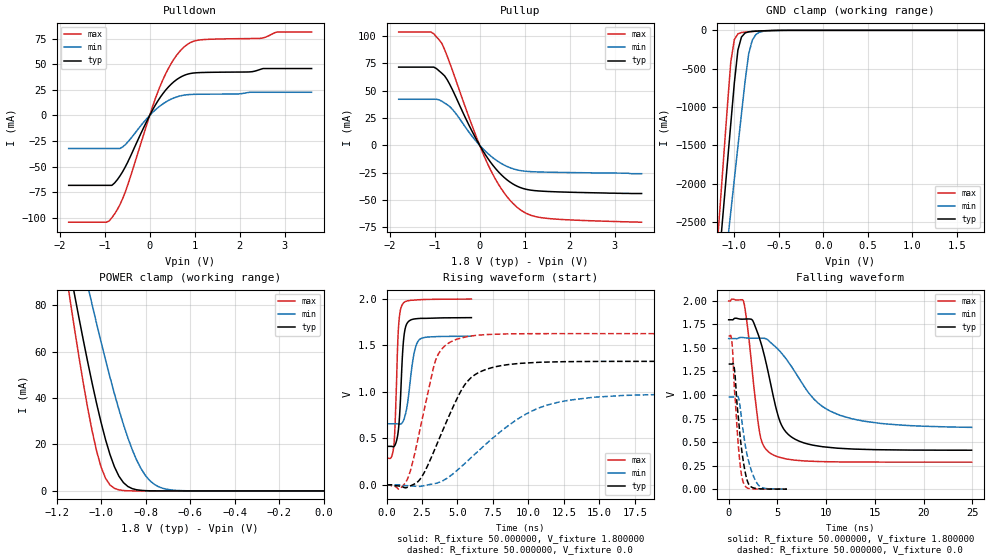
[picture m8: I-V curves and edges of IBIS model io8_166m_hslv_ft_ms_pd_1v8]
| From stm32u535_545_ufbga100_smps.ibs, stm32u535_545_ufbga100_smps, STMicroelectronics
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|   Model io8_166m_hslv_ft_ms_pd_1v8
[Model]  io8_166m_hslv_ft_ms_pd_1v8
Model_type I/O
Polarity   Non-Inverting
Enable   Active-Low
Vinl =   0.540000V
Vinh =   1.260000V
Vmeas =  0.900000V
Cref =   50.000000pF
Rref =   100.000000M
Vref =   0.0V
C_comp   3.358400pF   3.352800pF   3.400400pF
[Temperature Range]   25.000000   0.140000k   -40.000000
[Pullup Reference]   1.800000V   1.600000V   2.000000V
[Pulldown Reference]   0.0V   0.0V   0.0V
[POWER Clamp Reference]   1.800000V   1.600000V   2.000000V
[GND Clamp Reference]   0.0V   0.0V   0.0V
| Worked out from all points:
|   slope of the pulldown table from 0 to 0.27 V, typ, clamps not added: 13.6 ohm
|   slope of the pullup table from 0 to 0.27 V, typ, clamps not added: 15.9 ohm
|   GND clamp passes 1 mA (typ) near -0.50 V on its own axis
|   POWER clamp passes 1 mA (typ) near -0.86 V on its own axis
|   rising waveform, R_fixture 50.000000, V_fixture 1.800000: 20-80 % time 285ps typ, 490ps min, 232ps max; typ from 0.414 V to 1.8 V
|   rising waveform, R_fixture 50.000000, V_fixture 0.0: 20-80 % time 2.38ns typ, 4.83ns min, 1.41ns max; typ from 0 V to 1.33 V
|   falling waveform, R_fixture 50.000000, V_fixture 1.800000: 20-80 % time 1.98ns typ, 4.45ns min, 1.12ns max; typ from 1.8 V to 0.414 V
|   falling waveform, R_fixture 50.000000, V_fixture 0.0: 20-80 % time 792ps typ, 1.05ns min, 629ps max; typ from 1.33 V to 0 V
[Pulldown]
|Voltage   I(typ)   I(min)   I(max)
-1.8V     -68.38mA   -32.32mA   -104.4mA
-960mV    -68.38mA   -32.32mA   -104.4mA
-780mV    -66.08mA   -32.32mA   -96.43mA
-540mV    -50.22mA   -28.51mA   -74.66mA
0V        -10fA      -300fA     0A
240mV     18.04mA    9.6mA      29.42mA
480mV     30.68mA    16.02mA    50.95mA
780mV     39.48mA    19.99mA    67.56mA
1.14V     41.99mA    20.78mA    74.01mA
2.46V     45.09mA    22.69mA    75.45mA
2.82V     45.91mA    22.69mA    81.58mA
3.6V      45.91mA    22.69mA    81.58mA
[Pullup]
|Voltage   I(typ)   I(min)   I(max)
-1.8V     71.67mA    42.2mA     103.8mA
-1.08V    71.67mA    42.2mA     103.8mA
-840mV    66.04mA    40.35mA    93.41mA
-720mV    60.02mA    37.18mA    81.6mA
-600mV    50.51mA    32.72mA    68.09mA
-180mV    13.77mA    8.913mA    19.32mA
180mV     -11.9mA    -7.442mA   -17.26mA
480mV     -26.98mA   -16.65mA   -39.76mA
840mV     -37.65mA   -22.63mA   -57.07mA
1.08V     -40.74mA   -24.01mA   -63.22mA
1.44V     -42.19mA   -24.58mA   -66.73mA
3.6V      -44.2mA    -26mA      -70.5mA
[GND_clamp]
|Voltage   I(typ)   I(min)   I(max)
-1.8V     -9.908A    -9.683A    -9.994A
-1.2V     -3.383A    -4.084A    -2.934A
-1.16V    -2.841A    -3.655A    -2.294A
-1.12V    -2.299A    -3.226A    -1.656A
-1.04V    -1.218A    -2.369A    -414.2mA
-1V       -684.7mA   -1.941A    -119.2mA
-960mV    -257.2mA   -1.514A    -45.67mA
-920mV    -87.04mA   -1.089A    -28.94mA
-840mV    -19.36mA   -312.8mA   -18.98mA
-800mV    -13.56mA   -132.4mA   -15.51mA
-720mV    -8.053mA   -25.67mA   -9.505mA
1.8V      45.71uA    33.32uA    56.11uA
[POWER_clamp]
|Voltage   I(typ)   I(min)   I(max)
-1.8V     470.8mA    433.7mA    554.6mA
-1.14V    95.25mA    122.7mA    82.82mA
-1.12V    84.97mA    114mA      70.27mA
-1.06V    55.51mA    88.42mA    35.67mA
-1.04V    46.34mA    80.15mA    25.76mA
-1V       29.51mA    64.13mA    10.3mA
-940mV    10.39mA    41.86mA    1.109mA
-900mV    3.624mA    28.77mA    182.8uA
-840mV    490.7uA    13.24mA    11.35uA
-800mV    116.8uA    6.532mA    1.77uA
-740mV    13.2uA     1.724mA    109.3nA
0V        0A         18.75nA    0A
[Ramp]
| variable   typ   min   max
dV/dt_r  0.79734/2.37637n   0.58685/4.82328n   0.97632/1.40801n
dV/dt_f  0.83132/1.97334n   0.56144/4.43860n   1.02745/1.11951n
R_load = 50.000000
[Rising Waveform]
R_fixture= 50.000000
V_fixture= 1.800000
V_fixture_min= 1.600000
V_fixture_max= 2.000000
|time   V(typ)   V(min)   V(max)
0s        413.8mV    656.4mV    287.1mV
516.5ps   412.1mV    656.5mV    424.9mV
612.6ps   432.1mV    656.5mV    688.9mV
828.8ps   581mV      655.3mV    1.656V
1.093ns   1.307V     664.4mV    1.934V
1.213ns   1.578V     699.8mV    1.96V
1.369ns   1.712V     782.7mV    1.975V
1.886ns   1.783V     1.368V     1.988V
2.246ns   1.79V      1.551V     1.991V
5.982ns   1.8V       1.599V     2V
[Rising Waveform]
R_fixture= 50.000000
V_fixture= 0.0
V_fixture_min= 0.0
V_fixture_max= 0.0
|time   V(typ)   V(min)   V(max)
0s        -16.28uV   -2.051uV   -26.57uV
850.9ps   -12.33mV   244.4uV    -47.06mV
1.451ns   -27.91mV   -9.693mV   54.62mV
2.352ns   57.36mV    -17.03mV   590.9mV
3.453ns   401.2mV    15.04mV    1.338V
4.705ns   842.8mV    120.4mV    1.552V
5.656ns   1.106V     248.7mV    1.595V
6.757ns   1.227V     403.7mV    1.614V
11.56ns   1.322V     868.3mV    1.627V
24.92ns   1.329V     979.8mV    1.627V
[Falling Waveform]
R_fixture= 50.000000
V_fixture= 1.800000
V_fixture_min= 1.600000
V_fixture_max= 2.000000
|time   V(typ)   V(min)   V(max)
0s        1.8V       1.599V     2V
1.552ns   1.806V     1.609V     1.986V
2.452ns   1.794V     1.604V     1.221V
3.203ns   1.588V     1.604V     585.9mV
4.304ns   1.12V      1.558V     379.7mV
5.556ns   654.5mV    1.428V     329.7mV
7.658ns   493.6mV    1.106V     300.8mV
9.61ns    451.1mV    879.5mV    292.5mV
12.61ns   427mV      748.5mV    288.4mV
24.92ns   413.8mV    656.4mV    287.1mV
[Falling Waveform]
R_fixture= 50.000000
V_fixture= 0.0
V_fixture_min= 0.0
V_fixture_max= 0.0
|time   V(typ)   V(min)   V(max)
0s        1.329V     979.8mV    1.627V
324.3ps   1.329V     979.9mV    1.568V
420.4ps   1.334V     979.9mV    1.437V
552.6ps   1.302V     979.9mV    1.135V
1.093ns   649.3mV    930.4mV    343.6mV
1.297ns   448.4mV    773.1mV    162.1mV
1.514ns   287.7mV    598.5mV    68.23mV
2.078ns   49.23mV    283.4mV    6.605mV
3.027ns   4.831mV    45.48mV    1.211mV
5.982ns   -16.28uV   -2.051uV   -26.57uV
